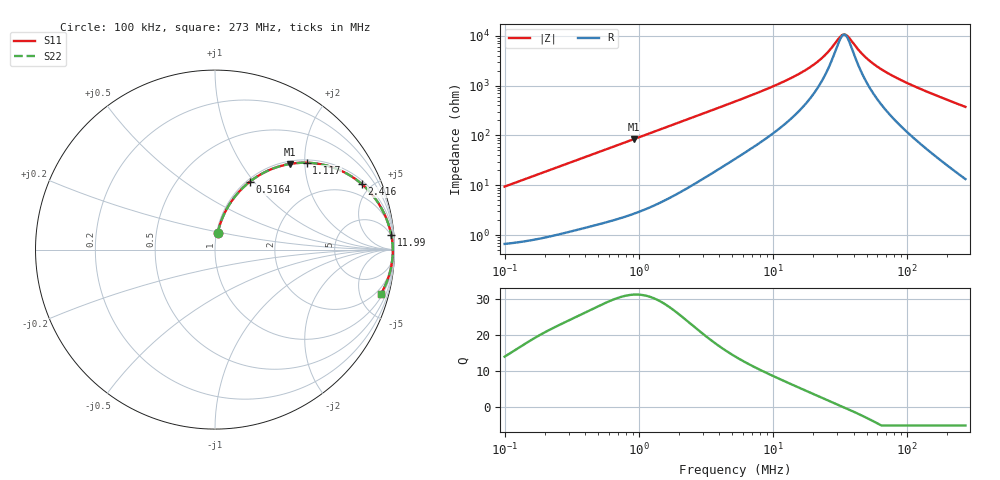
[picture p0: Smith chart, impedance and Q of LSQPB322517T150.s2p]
! LSQPB322517T150  S-PARAMETER MODEL  ( General Type )
! Model Generated by TAIYO YUDEN Corporation (http://www.ty-top.com)
! Version 2.0
! TAIYO YUDEN Control No. 100810NG22EB-FKC
! Copyright(c) 2009 TAIYO YUDEN CO.,LTD. All Rights Reserved.
! Product Description (link to TY-COMPAS)
! https://ds.yuden.co.jp/TYCOMPAS/or/detail?pn=LSQPB322517T150K&u=M
! Products Name : Inductors
! Characteristics :
!  Inductance : 15 uH , SRF(min) : 20 MHz , DC Resistance(max) : 0.684 Ohm
!  Rated Current : Saturation :700 mA , Temp Rise : 530 mA (40 degC)
!  Case Size : 3.2 x 2.5 / 0.126 x 0.098 [mm/inch] , Thickness : 1.7 / 0.068 [mm/inch]
!  (Conditions: Temperature = 25 degC , DC Bias Current/Voltage = 0A / 0V)
! External Node Assignments :
!  1  o---GGG---o  2
! GND o---------o GND
! Frequency Range : 0.1MHz  -  272.98108MHz  [ 402 STEP ]
# MHz S RI R 50
! Freq[MHz].  S11 Real  S11 Imag  S21 Real  S21 Imag  S12 Real  S12 Imag  S22 Real  S22 Imag
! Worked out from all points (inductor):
!   401 points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, 100 kHz to 273 MHz, reference 50 ohm
!   read as one part in series: L = 14.9 uH near 104 kHz
!   highest Q = 31.3 at 916.5 kHz (marker M1), where L = 14.6 uH
!   self-resonance near 33.54 MHz
!   S11 on the Smith chart (normalised r, x): 100 kHz: 1.01, +0.19; 516.4 kHz: 1.03, +0.95; 1.117 MHz: 1.07, +2.04; 2.416 MHz: 1.19, +4.40; 11.99 MHz: 4, +24; 273 MHz: 1.27, -7.49
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0.1  0.0152 0.092  0.9848 -0.092  0.9848 -0.092  0.0152 0.092
0.216283  0.0474 0.1906  0.9526 -0.1906  0.9526 -0.1906  0.0474 0.1906
0.376316  0.1175 0.3033  0.8825 -0.3033  0.8825 -0.3033  0.1175 0.3033
0.516413  0.193 0.3774  0.807 -0.3774  0.807 -0.3774  0.193 0.3774
0.916468  0.4158 0.4771  0.5842 -0.4771  0.5842 -0.4771  0.4158 0.4771
1.116916  0.5102 0.484  0.4898 -0.484  0.4898 -0.484  0.5102 0.484
1.416134  0.6218 0.4683  0.3782 -0.4683  0.3782 -0.4683  0.6218 0.4683
2.415702  0.8187 0.3644  0.1813 -0.3644  0.1813 -0.3644  0.8187 0.3644
3.44881  0.8959 0.2798  0.1041 -0.2798  0.1041 -0.2798  0.8959 0.2798
5.329134  0.9472 0.1907  0.0528 -0.1907  0.0528 -0.1907  0.9472 0.1907
11.99113  0.9823 0.0805  0.0177 -0.0805  0.0177 -0.0805  0.9823 0.0805
19.66158  0.9886 0.0379  0.0114 -0.0379  0.0114 -0.0379  0.9886 0.0379
24.92886  0.99 0.0209  0.01 -0.0209  0.01 -0.0209  0.99 0.0209
31.60723  0.9906 0.00487  0.00941 -0.00487  0.00941 -0.00487  0.9906 0.00487
34.20958  0.9907 -0.000365  0.00933 0.000365  0.00933 0.000365  0.9907 -0.000365
37.0262  0.9907 -0.00561  0.00932 0.00561  0.00932 0.00561  0.9907 -0.00561
44.24071  0.9905 -0.0176  0.00952 0.0176  0.00952 0.0176  0.9905 -0.0176
50.81061  0.9901 -0.0273  0.00991 0.0273  0.00991 0.0273  0.9901 -0.0273
60.711  0.9892 -0.0405  0.0108 0.0405  0.0108 0.0405  0.9892 -0.0405
73.9896  0.9877 -0.0567  0.0123 0.0567  0.0123 0.0567  0.9877 -0.0567
128.736  0.9773 -0.1151  0.0227 0.1151  0.0227 0.1151  0.9773 -0.1151
272.9811  0.9259 -0.2447  0.0741 0.2447  0.0741 0.2447  0.9259 -0.2447
